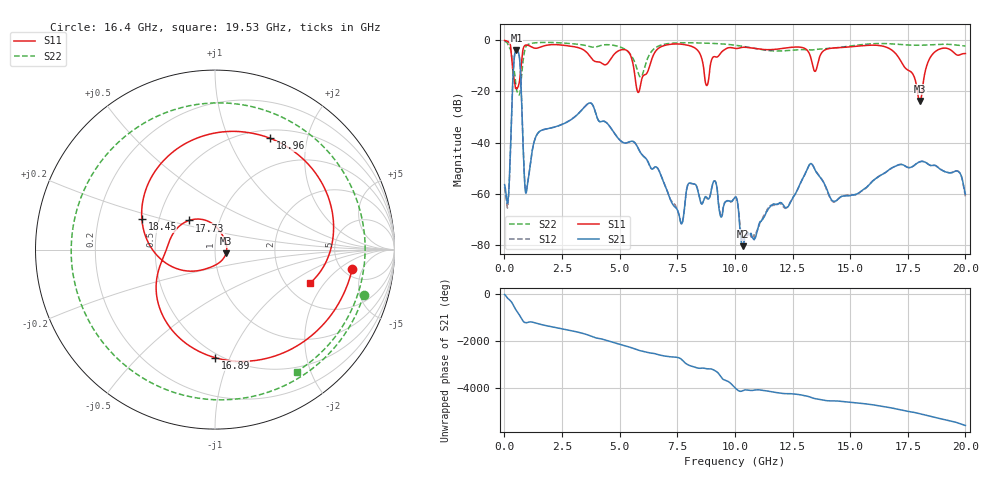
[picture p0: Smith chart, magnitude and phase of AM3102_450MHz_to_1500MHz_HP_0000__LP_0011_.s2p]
!Agilent Technologies,E8364B,MY43040894,A.07.50.67
!Agilent E8364B: A.07.50.67
!Date: Thursday, January 11, 2018 05:15:04
!Correction: S11(Full 2 Port(1,2))
!S21(Full 2 Port(1,2))
!S12(Full 2 Port(1,2))
!S22(Full 2 Port(1,2))
!S2P File: Measurements: S11, S21, S12, S22:
# Hz S  dB  R 50
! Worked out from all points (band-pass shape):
!   1601 points, 10 MHz to 20 GHz, reference 50 ohm
!   highest |S21| = -3.77 dB at 522.2 MHz (marker M1); lowest = -80.5 dB at 10.34 GHz (marker M2)
!   |S21| within 3 dB of the highest: 429.9 MHz to 654.4 MHz (224.5 MHz wide, 41.4 % of centre)
!   lowest |S11| = -23.7 dB at 18.03 GHz (marker M3), VSWR 1.14, Z = 56.5 - j2.31 ohm
!   |S11| at or under -10 dB: 347.1 MHz to 727.6 MHz (380.6 MHz wide, 70.8 % of centre); 5.596 GHz to 6.303 GHz (706.6 MHz wide, 11.9 % of centre); 17.32 GHz to 18.32 GHz (998 MHz wide, 5.6 % of centre)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
!   |S22| runs from -21.3 to -0.3 dB; largest |S21 - S12| = 0.0022
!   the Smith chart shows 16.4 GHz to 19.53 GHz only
!   S11 on the Smith chart (normalised r, x): 16.4 GHz: 5.97, -3.24; 16.89 GHz: 0.47, -0.88; 17.73 GHz: 0.71, +0.24; 18.45 GHz: 0.40, +0.17; 18.96 GHz: 0.60, +1.43; 19.53 GHz: 2.68, -1.46
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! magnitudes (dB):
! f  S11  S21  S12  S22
! 10 MHz  -0.1  -56.4  -57.4  -0.3
! 172.4 MHz  -0.6  -61.5  -62.5  -2.1
! 522.2 MHz  -18.8  -3.8  -3.8  -19.1
! 959.5 MHz  -1.9  -59.1  -58.6  -2.1
! 1.459 GHz  -3.0  -36.3  -36.2  -0.9
! 3.346 GHz  -3.3  -27.4  -27.4  -1.7
! 5.807 GHz  -20.4  -42.3  -42.3  -12.8
! 6.682 GHz  -3.1  -50.5  -50.5  -2.3
! 7.669 GHz  -1.5  -71.7  -71.8  -1.0
! 8.781 GHz  -17.7  -61.5  -61.7  -1.1
! 10.01 GHz  -3.2  -61.5  -61.4  -1.9
! 10.34 GHz  -2.7  -80.5  -78.7  -2.4
! 13.34 GHz  -8.5  -48.4  -48.4  -3.8
! 16.4 GHz  -2.2  -52.4  -52.4  -1.2
! 16.68 GHz  -3.1  -50.7  -50.7  -1.3
! 16.89 GHz  -4.4  -49.6  -49.5  -1.4
! 17.73 GHz  -13.3  -49.3  -49.3  -1.9
! 18.03 GHz  -23.7  -47.5  -47.5  -1.9
! 18.45 GHz  -7.1  -48.8  -48.8  -1.8
! 18.96 GHz  -3.2  -50.7  -50.7  -1.6
! 19.53 GHz  -5.0  -51.3  -51.2  -1.7
! 20 GHz  -5.2  -60.2  -61.0  -2.3
